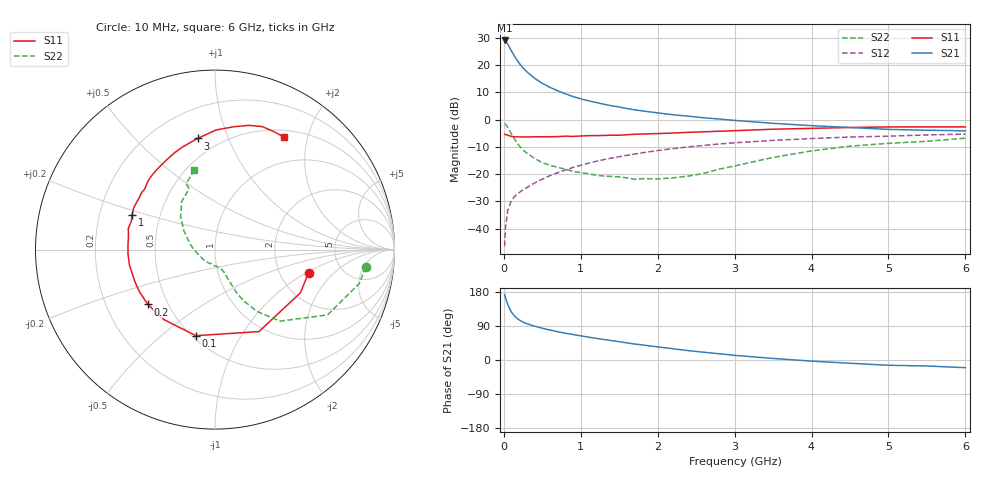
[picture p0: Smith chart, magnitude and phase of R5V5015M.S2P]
! SIEMENS Small Signal Semiconductors
! BFR183
! Si NPN RF Bipolar Junction Transistor in SOT23
! VCE = 0.5 V  IC = 15 mA
! Common Emitter S-Parameters:  May  1996
# GHz  S  MA  R  50
!  f  S11  S21  S12  S22
! GHz  MAG  ANG  MAG  ANG  MAG  ANG  MAG  ANG
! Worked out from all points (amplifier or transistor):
!   36 points, 10 MHz to 6 GHz, reference 50 ohm
!   highest |S21| = 29.0 dB at 10 MHz (marker M1)
!   |S21| within 3 dB of that: start of sweep to 83.05 MHz
!   unconditionally stable (mu >= 1): 354.9 MHz to end of sweep
!   at 250 MHz: K = 0.87, MSG = 22.3 dB, |S12| = -25.7 dB
!   at 1.4 GHz: K = 1.18, MAG = 7.0 dB, |S12| = -14.1 dB
!   at 6 GHz: K = 1.04, MAG = -0.6 dB, |S12| = -5.3 dB
!   S11 on the Smith chart (normalised r, x): 10 MHz: 2.90, -1.04; 100 MHz: 0.52, -0.66; 200 MHz: 0.39, -0.31; 1 GHz: 0.34, +0.18; 3 GHz: 0.38, +0.78; 6 GHz: 0.60, +1.63
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0.01  0.5368 -13.8  28.2 172.7  0.0048 81.0  0.8443 -6.6
0.02  0.5336 -26.8  27.59 165.4  0.0101 78.4  0.8262 -13.2
0.05  0.5183 -61.8  24.37 146.8  0.0215 67.0  0.7254 -30.1
0.1  0.4913 -102.5  18.03 126.1  0.0333 57.5  0.539 -47.7
0.15  0.4826 -126.0  13.64 113.4  0.0405 54.1  0.4155 -55.9
0.2  0.4833 -140.8  10.77 105.6  0.0461 54.1  0.3311 -60.5
0.25  0.4818 -150.8  8.842 99.9  0.0518 55.1  0.2763 -63.2
0.3  0.4808 -158.1  7.508 95.7  0.0571 57.0  0.2436 -63.9
0.4  0.4843 -169.6  5.723 89.1  0.0691 59.0  0.1943 -65.6
0.5  0.4853 -177.2  4.61 83.7  0.0811 60.8  0.1623 -66.8
0.6  0.4856 176.5  3.902 79.1  0.0941 61.5  0.1458 -67.3
0.7  0.4878 171.1  3.382 74.7  0.1063 61.8  0.1337 -68.4
0.8  0.4972 166.3  2.969 70.8  0.1194 61.5  0.1234 -70.0
1  0.501 157.1  2.405 63.7  0.1461 60.7  0.1066 -75.3
1.1  0.5084 153.2  2.212 60.3  0.159 60.0  0.1019 -79.6
1.7  0.5386 132.5  1.509 42.1  0.2343 53.1  0.0805 -105.3
2.2  0.5675 118.5  1.226 29.6  0.2938 46.0  0.0857 -141.0
3  0.627 98.9  0.967 12.3  0.3761 33.9  0.1414 167.6
3.5  0.6668 89.4  0.855 4.1  0.4164 26.3  0.2029 148.9
4.5  0.7174 74.8  0.717 -8.6  0.4802 12.4  0.3267 124.5
5.5  0.7347 63.5  0.639 -15.8  0.5248 1.5  0.401 113.6
6  0.7349 58.4  0.623 -20.3  0.5425 -5.7  0.4567 104.8
